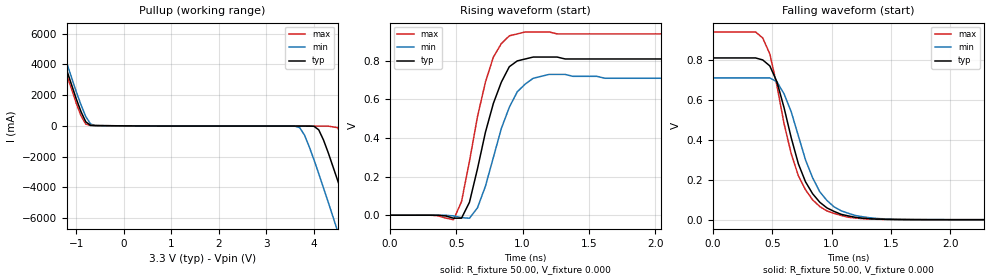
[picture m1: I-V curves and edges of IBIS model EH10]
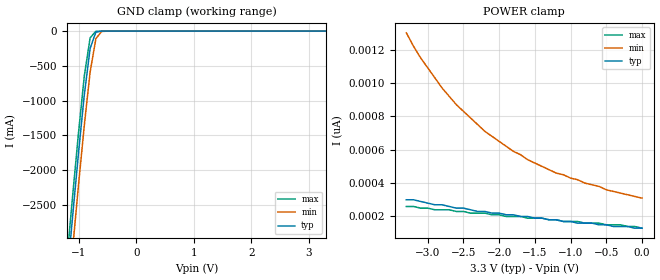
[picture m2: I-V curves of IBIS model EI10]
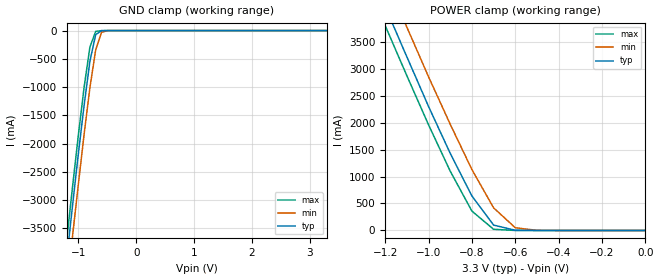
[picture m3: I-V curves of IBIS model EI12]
|   * 9db1200c.ibs * IBIS 2.1 Model file
| Rev History
| Rev No.   Description
| 1.0   Initial release with Updated Parasitic Parameters
| 1.1   Corrected diff table  Dec 15, 2009
| 1.2   Added Vmeas, Vref and Rref to models EH10 and EIOD1 lfp
| 1.3   Corrected diff table Feb 17, 2012 lfp
[IBIS Ver]   2.1
[Comment char]  |_char
[File name]   9db1200c.ibs
[Date]   Feb 17, 2012
[File Rev]   1.3
[Source]   Originated at Integrated Circuit Systems, Inc.
[Disclaimer] (C) Copyright Integrated Circuit Systems, Inc. 2005
   All rights reserved
ICS hereby grants the user of this IBIS model a non-exclusive,
nontransferable license to use this IBIS model under the following terms.
Before using this IBIS model, the user should read this license.
If the user does not accept these terms,  the IBIS model should be
returned to ICS within 30 days.
   The user is granted this license only to use the IBIS model and
is not granted rights to sell, load, rent, lease or license the IBIS
model in whole or in part, or in modified form to anyone other than
user. User may modify the IBIS model to suit its specific
applications but rights to derivative works and such modifications
shall belong to ICS.
   This IBIS model is provided on an "AS IS" basis and ICS makes
absolutely no warranty with respect to the information contained
herein. ICS DISCLAIMS AND CUSTOMER WAIVES ALL WARRANTIES, EXPRESS
OR IMPLIED, INCLUDING WARRANTIES OF MERCHANTABILITY OR FITNESS FOR
A PARTICULAR PURPOSE. The entire risk as to quality and performance
is with the Customer. ACCORDINGLY, IN NO EVENT SHALL THE COMPANY BE
LIABLE FOR ANY DAMAGES, WHETHER IN CONTRACT OR TORT,INCLUDING ANY
LOST PROFITS OR OTHER INCIDENTAL, CONSEQUENTIAL, EXEMPLARY, OR
PUNITIVE DAMAGES ARISING OUT OF THE USE OR APPLICATION OF THE IBIS
model provided in this package. Further, ICS reserves the right to
make changes without notice to any product herein to improve
reliability, function, or design. ICS does not convey any license
under patent rights or any other intellectual property rights,
including those of third parties.
   ICS is not obligated to provide maintenance or support
for the licensed IBIS model.
|   COMPONENT: ICS9DB1200
[Component]   ICS9DB1200
[Manufacturer]  ICS
[Package]
| variable   typ   min   max
R_pkg   81.1m   62.2m   100.0m
L_pkg   6.7nH   4.9nH   8.5nH
C_pkg   0.53pF  0.21pF  0.85pF
[Pin]   signal_name   model_name   R_pin   L_pin   C_pin
1   VDD   POWER
2   DIF_IN   EI22
3   DIF_IN#   EI22
4   GND   GND
5   OE0#   EI8
6   DIF_0   EH10
7   DIF_0#   EH10
8   VDD   POWER
9   GND   GND
10   OE1#   EI8
11   DIF_1   EH10
12   DIF_1#   EH10
13   OE2#   EI8
14   DIF_2   EH10
15   DIF_2#   EH10
16   GND   GND
17   VDD   POWER
18   OE3#   EI8
19   DIF_3   EH10
20   DIF_3#   EH10
21   OE4#   EI8
22   DIF_4   EH10
23   DIF_4#   EH10
24   VDD   POWER
25   GND   GND
26   OE5#   EI8
27   DIF_5   EH10
28   DIF_5#   EH10
29   ADR_SEL   EI12
30   HIGH_BW#   EI10
31   FS2   EI12
32   SMBCLK   EI8
33   SMBDAT   EIOD1
34   FS1   EI12
35   BYPASS#/PLL   EI10
36   PWRGD#/PD   EI8
37   DIF_6#   EH10
38   DIF_6   EH10
39   OE6#   EI8
40   GND   GND
41   VDD   POWER
42   DIF_7#   EH10
43   DIF_7   EH10
44   OE7#   EI8
45   DIF_8#   EH10
46   DIF_8   EH10
47   OE8#   EI8
48   VDD   POWER
49   GND   GND
50   DIF_9#   EH10
51   DIF_9   EH10
52   OE9#   EI8
53   DIF_10#   EH10
54   DIF_10   EH10
55   OE10#   EI8
56   GND   GND
57   VDD   POWER
58   DIF_11#   EH10
59   DIF_11   EH10
60   OE11#   EI8
61   FS0   EI12
62   IREF   EI5
63   GNDA   GND
64   VDDA   POWER
|* Either 3.3V or 2.5V
|** All model are simulated with typical corner process
[Diff Pin]   inv_pin   vdiff   tdelay_typ
2   3   NA   NA
6   7   NA   NA
11   12   NA   NA
14   15   NA   NA
19   20   NA   NA
22   23   NA   NA
27   28   NA   NA
38   37   NA   NA
43   42   NA   NA
46   45   NA   NA
51   50   NA   NA
54   53   NA   NA
59   58   NA   NA
| Models and submodels in the file (7): EH10 (Open_source), EI10 (Input), EI12 (Input), EI22 (Input), EI5 (Input), EI8 (Input), EIOD1 (I/O_open_drain)
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|   Model EH10
[Model]   EH10
Model_type   Open_source
Polarity   Inverting
Vmeas = 0.35V
Cref =   2.00pF
Rref =  500
Vref =   0.0V
C_comp   3.40pF   2.85pF   3.95pF
[Temperature Range]   27.00   70.00   0.000
[Voltage Range]   3.30V   3.00V   3.70V
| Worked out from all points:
|   slope of the pullup table from 0 to 0.495 V, typ, clamps not added: 52.5 ohm
|   rising waveform, R_fixture 50.00, V_fixture 0.000: 20-80 % time 184ps typ, 190ps min, 175ps max; typ from 0 V to 0.81 V
|   falling waveform, R_fixture 50.00, V_fixture 0.000: 20-80 % time 249ps typ, 257ps min, 238ps max; typ from 0.81 V to 0 V
[Pullup]
| voltage   I(typ)   I(min)   I(max)
-3.3V     24.1A      24.53A     23.84A
-1.5V     6.41A      6.88A      6.12A
-1V       1.75A      2.21A      1.46A
-800mV    260mA      600mA      110mA
-600mV    15.73mA    18.78mA    16.94mA
3.7V      -16.24mA   -120mA     -18.9mA
4.1V      -260mA     -3.11A     -18.93mA
4.5V      -3.57A     -6.88A     -120mA
4.7V      -5.46A     -8.8A      -1.47A
4.9V      -7.38A     -10.74A    -3.28A
5.3V      -11.26A    -14.65A    -7.09A
6.6V      -24.07A    -27.46A    -19.85A
[Ramp]
| variable   typ   min   max
dV/dt_r   0.48/0.18n   0.43/0.19n   0.56/0.17n
dV/dt_f   0.48/0.24n   0.43/0.25n   0.56/0.23n
R_load = 50.00
[Rising Waveform]
R_fixture = 50.00
V_fixture = 0.000
V_fixture_min = 0.000
V_fixture_max = 0.000
| time   V(typ)   V(min)   V(max)
0s        0V         0V         0V
480ps     -15.47mV   -3.46mV    -23.12mV
540ps     -15.3mV    -12.64mV   70.54mV
600ps     67.36mV    -15.53mV   280mV
660ps     240mV      38.03mV    510mV
780ps     580mV      300mV      820mV
900ps     770mV      560mV      930mV
1.02ns    810mV      680mV      950mV
1.2ns     820mV      730mV      950mV
3ns       810mV      710mV      940mV
[Falling Waveform]
R_fixture = 50.00
V_fixture = 0.000
V_fixture_min = 0.000
V_fixture_max = 0.000
| time   V(typ)   V(min)   V(max)
0s        810mV      710mV      940mV
420ps     800mV      710mV      910mV
480ps     770mV      710mV      830mV
540ps     690mV      690mV      670mV
600ps     560mV      630mV      480mV
720ps     280mV      420mV      220mV
840ps     130mV      210mV      99.4mV
960ps     59.19mV    96.59mV    44.14mV
1.38ns    3mV        6.11mV     2.11mV
3ns       8.4uV      8.96uV     9.06uV
|   Model EI10
[Model]   EI10
Model_type   Input
Polarity   Non-Inverting
Enable   Active-High
Vinl =   0.80V
Vinh =   2.00V
C_comp   5.50pF   5.00pF   6.00pF
[Temperature Range]   27.00   70.00   0.000
[Voltage Range]   3.30V   3.00V   3.70V
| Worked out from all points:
|   GND clamp passes 1 mA (typ) near -0.60 V on its own axis
[GND_clamp]
| voltage   I(typ)   I(min)   I(max)
-3.3V     -24.05A    -24.49A    -23.79A
-1.2V     -3.55A     -4.02A     -3.26A
-1.1V     -2.63A     -3.1A      -2.34A
-1V       -1.74A     -2.2A      -1.45A
-900mV    -910mA     -1.35A     -640mA
-800mV    -250mA     -590mA     -96.82mA
-700mV    -14.58mA   -110mA     -3.87mA
-600mV    -880uA     -5.82mA    -450uA
-500mV    -88.5uA    -350uA     -45.09uA
3.3V      130pA      340pA      120pA
[POWER_clamp]
| voltage   I(typ)   I(min)   I(max)
-3.3V     300pA      1.3nA      260pA
-3.1V     290pA      1.15nA     250pA
-2.9V     270pA      1.03nA     240pA
-2.8V     270pA      970pA      240pA
-2.6V     250pA      870pA      230pA
-2.2V     230pA      710pA      220pA
-1.8V     210pA      590pA      200pA
-1.2V     180pA      460pA      180pA
-900mV    160pA      420pA      170pA
-500mV    150pA      360pA      150pA
-300mV    140pA      340pA      150pA
0V        130pA      310pA      130pA
|   Model EI12
[Model]   EI12
Model_type   Input
Polarity   Inverting
Vinl =   0.80V
Vinh =   2.00V
C_comp   2.00pF   1.50pF   2.50pF
[Temperature Range]   27.00   70.00   0.000
[Voltage Range]   3.30V   3.00V   3.70V
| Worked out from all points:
|   GND clamp passes 1 mA (typ) near -0.54 V on its own axis
|   POWER clamp passes 1 mA (typ) near -0.53 V on its own axis
[GND_clamp]
| voltage   I(typ)   I(min)   I(max)
-3.3V     -24.55A    -25.06A    -24.24A
-1.2V     -4.03A     -4.56A     -3.69A
-1.1V     -3.09A     -3.63A     -2.76A
-1V       -2.18A     -2.72A     -1.85A
-900mV    -1.32A     -1.83A     -1A
-800mV    -540mA     -1.01A     -290mA
-700mV    -71.85mA   -340mA     -14.4mA
-600mV    -2.26mA    -32.39mA   -430uA
-500mV    -85.89uA   -1.3mA     -27.21uA
3.3V      71.48pA    2.74uA     48.84pA
[POWER_clamp]
| voltage   I(typ)   I(min)   I(max)
-3.3V     24.69A     25.21A     24.36A
-1.2V     4.15A      4.71A      3.8A
-1.1V     3.22A      3.77A      2.87A
-1V       2.3A       2.85A      1.96A
-900mV    1.43A      1.97A      1.1A
-800mV    640mA      1.13A      360mA
-700mV    100mA      420mA      21.87mA
-600mV    3.35mA     50.54mA    380uA
-500mV    78.94uA    2.11mA     5.9uA
0V        71.48pA    320pA      74.52pA
